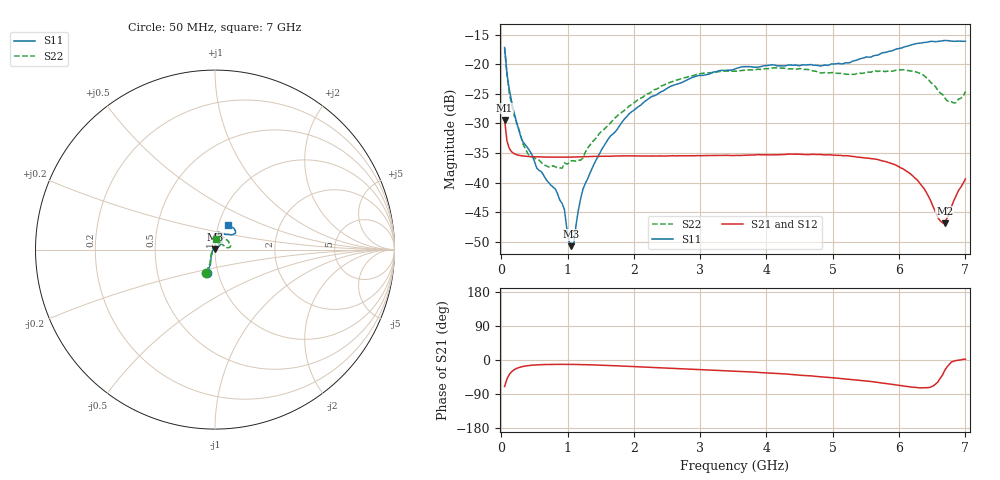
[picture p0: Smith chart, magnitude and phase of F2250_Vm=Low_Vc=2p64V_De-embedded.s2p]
! Integrated Device Technology
! Corporate Headquarters
! 6024 Silver Creek Valley Road
! San Jose, CA 95138  USA
! Phone:  1-408-284-8200
! Toll Free:  1-800-223-1366
! Webpage:  http://www.idt.com/
! Timing and RF Division
! 515 Groton Road, Suite 102
! Westford, MA 01886-6024
! Device:  F2250
! Description: Voltage Variable RF Attenuator
! Frequency:  50.0 -  6000.00 MHz
! Package:  3x3 mm Thin QFN Plastic Package: 16 pin
! Ports:  2 RF, 3 DC
!  Pin  1  = GND
!  Pin  2  = NC
!  Pin  3  = RF1  = Port 1
!  Pin  4  = NC
!  Pin  5  = GND
!  Pin  6  = GND
!  Pin  7  = GND
!  Pin  8  = GND
!  Pin  9  = NC
!  Pin 10  = RF2  = Port 2
!  Pin 11  = NC
!  Pin 12  = GND
!  Pin 13  = GND
!  Pin 14  = VCNTRL
!  Pin 15  = VDD
!  Pin 16  = VMODE
! Vcntrl:  2.640 Volts
! Vmode:  +0.000 Volts
! Vdd:  +3.30  Volts
! Current:  1.175 mA
! Data:  The device was measured on a the F2250 evaluation board which has
!  individual transmission lines to the RF pins.  Data was collected
!  using a calibrated network analyzer.  The evaluation board was
!  de-embedded using a TRL calibration technique.
!  The reference plane is the edge of the package pin.
! Misc:  SN 10
!  Action Tracker AT0258
! Date Measured:  2014-11-26
! Date:  2015-10-15  MJV
! Note:
!  Integrated Device Technology supplies this data as a sample of measured
!  data at the package pin for this product.  Your particular data for this
!  product may vary.
!  Data was taken at 25 degrees C.
!  Integrated Device Technology reserves the right to change this data at anytime.
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# GHz S dB R 50
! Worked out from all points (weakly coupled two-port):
!   201 points, 50 MHz to 7 GHz, reference 50 ohm
!   highest |S21| = -29.41 dB at 50 MHz (marker M1); lowest = -46.9 dB at 6.687 GHz (marker M2)
!   lowest |S11| = -50.7 dB at 1.058 GHz (marker M3), VSWR 1.01, Z = 49.8 + j0.241 ohm
!   |S11| at or under -10 dB: start of sweep to end of sweep
!   |S22| runs from -37.5 to -17.3 dB; largest |S21 - S12| = 7.5e-05
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0.05  -17.18 -108.6  -29.41 -69.8  -29.41 -69.8  -17.27 -111.0
0.08475  -21.45 -107.4  -32.92 -50.3  -32.91 -50.3  -21.75 -110.1
0.15425  -26.23 -116.6  -34.76 -31.2  -34.76 -31.1  -26.81 -122.4
0.29325  -32.22 -127.8  -35.43 -18.5  -35.43 -18.5  -32.10 -137.3
0.3975  -34.10 -141.8  -35.56 -15.0  -35.56 -15.0  -35.05 -160.3
0.5365  -37.56 -155.5  -35.63 -12.8  -35.63 -12.8  -36.06 177.9
0.91875  -43.50 157.9  -35.68 -11.5  -35.69 -11.5  -37.54 133.5
0.9535  -44.62 170.0  -35.68 -11.5  -35.69 -11.5  -36.65 131.1
1.023  -49.94 143.6  -35.68 -11.6  -35.68 -11.6  -36.64 115.9
1.05775  -50.70 124.1  -35.67 -11.6  -35.67 -11.6  -36.28 110.6
1.0925  -50.39 89.5  -35.66 -11.7  -35.66 -11.7  -36.30 106.5
1.162  -44.66 56.8  -35.64 -11.9  -35.64 -11.9  -36.21 95.4
1.2315  -41.11 44.1  -35.61 -12.1  -35.61 -12.1  -35.82 85.7
1.6485  -32.10 42.0  -35.52 -14.6  -35.52 -14.6  -29.87 64.6
2.37825  -24.87 47.4  -35.48 -20.3  -35.48 -20.3  -23.99 56.8
3.525  -20.80 72.5  -35.41 -29.5  -35.41 -29.5  -21.19 74.8
4.7065  -20.17 72.4  -35.20 -42.6  -35.20 -42.6  -21.14 72.3
5.85325  -17.81 40.4  -36.64 -63.3  -36.64 -63.3  -21.13 23.0
6.27025  -16.50 40.0  -39.50 -72.6  -39.50 -72.7  -21.36 9.6
6.68725  -15.99 48.8  -46.85 -27.7  -46.83 -27.4  -25.65 28.5
6.861  -16.13 55.1  -42.18 -1.3  -42.13 -1.3  -26.46 57.9
7  -16.13 63.2  -39.35 1.9  -39.31 1.7  -24.62 83.1
